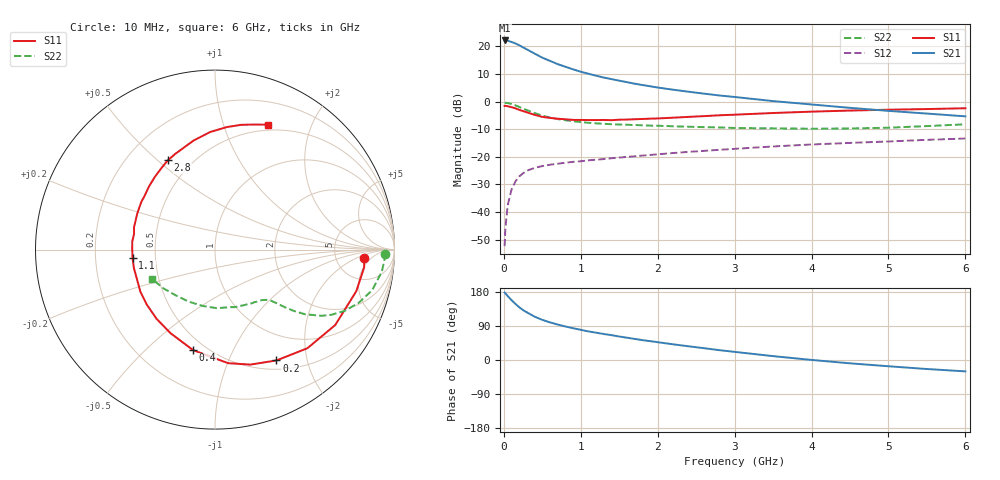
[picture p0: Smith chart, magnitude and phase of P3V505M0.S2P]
! SIEMENS Small Signal Semiconductors
! BFP181
! Si NPN RF Bipolar Junction Transistor in SOT143
! VCE = 0.5 V  IC = 5 mA
! Common Emitter S-Parameters:  March  1996
# GHz  S  MA  R  50
!  f  S11  S21  S12  S22
! GHz  MAG  ANG  MAG  ANG  MAG  ANG  MAG  ANG
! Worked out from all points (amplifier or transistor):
!   36 points, 10 MHz to 6 GHz, reference 50 ohm
!   highest |S21| = 22.1 dB at 10 MHz (marker M1)
!   |S21| within 3 dB of that: start of sweep to 283.3 MHz
!   unconditionally stable (mu >= 1): 873.9 MHz to end of sweep
!   at 250 MHz: K = 0.35, MSG = 22.8 dB, |S12| = -26.0 dB
!   at 1.4 GHz: K = 1.36, MAG = 10.7 dB, |S12| = -20.5 dB
!   at 6 GHz: K = 1.52, MAG = -0.2 dB, |S12| = -13.4 dB
!   S11 on the Smith chart (normalised r, x): 10 MHz: 10, -3; 200 MHz: 0.62, -1.52; 400 MHz: 0.43, -0.71; 1.1 GHz: 0.37, -0.04; 2.8 GHz: 0.37, +0.54; 6 GHz: 0.44, +1.41
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0.01  0.8315 -3.3  12.76 177.9  0.0024 85.3  0.9498 -1.4
0.02  0.8371 -6.7  12.73 175.9  0.0051 81.8  0.9467 -3.0
0.05  0.8207 -16.4  12.62 168.7  0.0132 82.2  0.9378 -7.5
0.1  0.7908 -32.1  11.99 158.0  0.0254 71.9  0.9044 -14.5
0.15  0.7529 -46.9  11.26 148.1  0.0355 63.9  0.8533 -20.4
0.2  0.7061 -61.0  10.47 139.2  0.0439 58.4  0.7989 -25.3
0.25  0.6703 -72.9  9.541 131.6  0.0502 53.0  0.7439 -29.2
0.3  0.6371 -83.4  8.786 125.7  0.0559 49.3  0.6981 -31.9
0.4  0.5734 -102.3  7.372 114.4  0.0628 43.1  0.6174 -35.7
0.5  0.5275 -118.0  6.226 105.9  0.0678 39.0  0.5557 -37.9
0.6  0.5047 -130.2  5.442 99.2  0.0716 36.7  0.5116 -39.3
0.7  0.488 -141.3  4.753 93.6  0.0747 35.1  0.4806 -40.2
0.9  0.4649 -159.2  3.825 83.9  0.0808 33.4  0.4405 -41.6
1.1  0.4618 -174.2  3.182 75.4  0.0861 32.6  0.4118 -43.2
1.3  0.4631 174.4  2.715 68.6  0.0907 32.0  0.3949 -45.2
1.7  0.4774 155.1  2.105 55.6  0.1018 31.9  0.375 -50.1
2.2  0.5094 136.1  1.637 41.4  0.1166 30.4  0.3562 -58.5
2.8  0.5629 117.8  1.287 26.0  0.1335 28.0  0.3394 -70.8
3.5  0.6193 101.1  1.018 10.2  0.1535 24.1  0.3265 -88.2
4.5  0.6858 84.5  0.768 -8.8  0.1781 16.7  0.3248 -116.8
5.5  0.7302 72.6  0.605 -23.8  0.2022 10.3  0.3591 -142.9
6  0.7551 67.2  0.539 -30.0  0.2138 6.5  0.3865 -154.8
